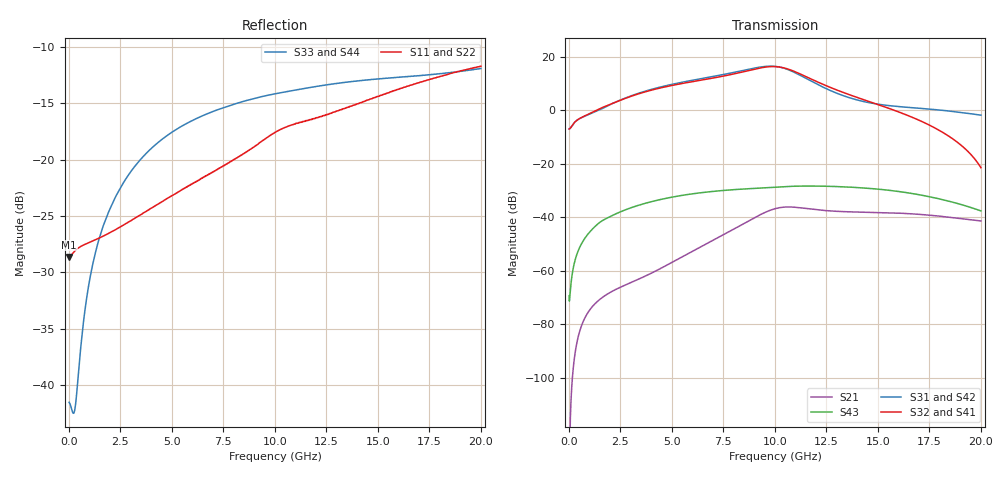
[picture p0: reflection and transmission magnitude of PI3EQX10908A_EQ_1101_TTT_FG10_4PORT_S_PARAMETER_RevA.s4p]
! NPort=4 DATA=2000 NOISE=0 GROUPDELAY=0 COMPLEX_DATAFORMAT=POLAR
! NumOfBlock=1 NumOfParam=0
! .MODEL Smodel S TSTONEFILE=PI3EQX10908A_EQ_1101_TTT_FG10_4PORT_S_PARAMETER_RevA.s4p TYPE=S
!  -- The above .MODEL line can be used for the S element in the netlist.
! The s parameter is extracted from the linear redriver, it is not bi-directional; only s(4,1)s(4,2) and s(3,1)s(3,2)
! should be the insertion loss
!Port definition:
!Port1 = input+
!Port2 = input-
!Port3 = output+
!Port4 = output-
# Hz S MA R  50
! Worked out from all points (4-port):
!   2000 points, 10 MHz to 20 GHz, reference 50 ohm
!   strongest paths, dB at 10 MHz, 5.01 GHz, 10.01 GHz, 15.01 GHz, 20 GHz:
!     S32: -6.9, 9.4, 16.4, 2.2, -21.4
!     S41: -6.9, 9.4, 16.4, 2.2, -21.4
!     S31: -6.9, 9.8, 16.5, 2.3, -1.8
!     S42: -6.9, 9.8, 16.5, 2.3, -1.8
!     S43: -69.4, -32.4, -28.7, -29.5, -37.6
!     S21: -127.2, -56.9, -36.8, -38.2, -41.4
!   lowest |S11| = -28.6 dB at 10 MHz (marker M1), VSWR 1.08, Z = 46.4 - j0.024 ohm
!   |S11| at or under -10 dB: start of sweep to end of sweep
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1e7  0.03701 -179.6  4.34e-07 14.6  0 0.0  0 0.0
     4.34e-07 14.6  0.03701 -179.6  0 0.0  0 0.0
     0.4506 1.2  0.4506 -178.8  0.008374 26.0  0.00034 -27.1
     0.4506 -178.8  0.4506 1.2  0.00034 -27.1  0.008374 26.0
6.46e9  0.08273 -120.9  0.002885 133.3  3.14e-07 67.7  1.728e-07 139.1
        0.002885 133.3  0.08276 -120.9  1.728e-07 139.1  3.14e-07 67.7
        3.969 -49.1  3.721 124.6  0.1563 14.4  0.029 19.4
        3.721 124.6  3.969 -49.1  0.029 19.4  0.1563 14.4
8.99e9  0.114 -112.1  0.009723 109.3  2.241e-06 22.0  1.414e-06 114.3
        0.009725 109.3  0.1141 -112.1  1.414e-06 114.3  2.241e-06 22.0
        6.201 -111.5  5.917 62.8  0.187 -5.7  0.03474 -6.9
        5.917 62.8  6.202 -111.5  0.03474 -6.9  0.187 -5.7
1.028e10  0.1364 -112.2  0.01524 72.1  4.01e-06 -12.5  4.206e-06 80.7
          0.01524 72.1  0.1364 -112.2  4.207e-06 80.7  4.01e-06 -12.5
          6.43 -165.1  6.456 8.4  0.1983 -14.5  0.03719 -20.0
          6.457 8.4  6.431 -165.1  0.03719 -20.0  0.1983 -14.5
1.141e10  0.1478 -113.5  0.01478 41.0  4.985e-06 -23.3  7.42e-06 44.2
          0.01478 41.0  0.1478 -113.5  7.422e-06 44.2  4.984e-06 -23.3
          4.183 153.2  4.485 -36.5  0.2069 -21.0  0.03843 -33.4
          4.485 -36.5  4.183 153.2  0.03843 -33.4  0.2069 -21.0
1.36e10  0.1712 -111.9  0.01267 13.7  1.366e-05 -36.0  1.633e-05 -5.6
         0.01266 13.8  0.1713 -111.9  1.633e-05 -5.6  1.365e-05 -36.0
         1.741 122.7  1.984 -84.5  0.2216 -32.5  0.03679 -60.0
         1.984 -84.4  1.741 122.7  0.03679 -60.0  0.2216 -32.5
2e10  0.2601 -114.9  0.008546 -39.9  8.834e-05 -148.0  7.171e-05 -139.3
      0.008542 -39.7  0.2602 -114.9  7.172e-05 -139.3  8.833e-05 -148.0
      0.816 53.1  0.08499 169.4  0.2539 -52.2  0.01318 -136.5
      0.08532 169.8  0.8167 53.1  0.01317 -136.5  0.2539 -52.2
